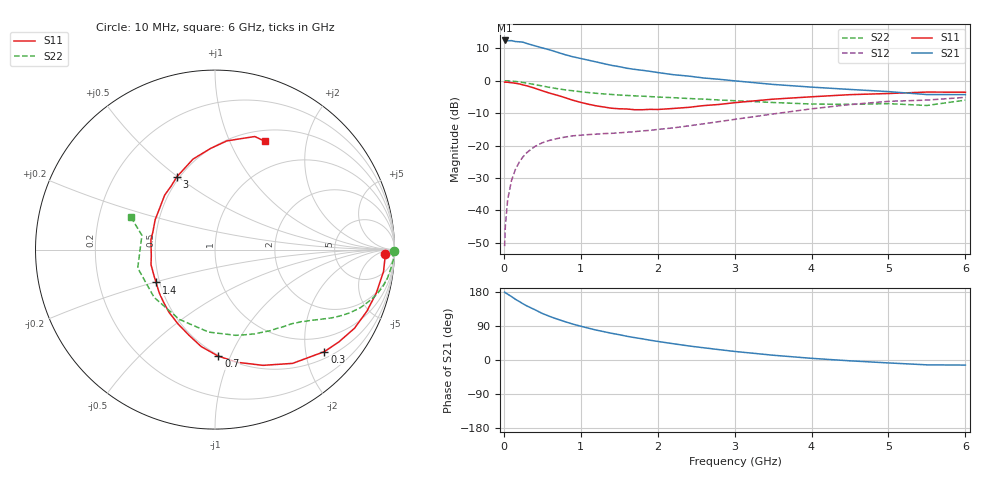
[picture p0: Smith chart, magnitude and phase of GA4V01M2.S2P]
! Infineon Technologies  Discrete & RF Semiconductors
! BF775
! Si NPN RF Bipolar Junction Transistor in SOT23
! VCE = 4 V  IC = 1.2 mA
! Common Emitter S-Parameters:  May  1996
# GHz  S  MA  R  50
!  f  S11  S21  S12  S22
! GHz  MAG  ANG  MAG  ANG  MAG  ANG  MAG  ANG
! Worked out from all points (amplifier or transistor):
!   36 points, 10 MHz to 6 GHz, reference 50 ohm
!   highest |S21| = 12.4 dB at 10 MHz (marker M1)
!   |S21| within 3 dB of that: start of sweep to 609.4 MHz
!   unconditionally stable (mu >= 1): 1.361 GHz to 3.872 GHz; 5.166 GHz to end of sweep
!   at 250 MHz: K = 0.22, MSG = 17.7 dB, |S12| = -23.5 dB
!   at 1.4 GHz: K = 1.03, MAG = 9.5 dB, |S12| = -16.2 dB
!   at 6 GHz: K = 1.01, MAG = -0.2 dB, |S12| = -5.1 dB
!   S11 on the Smith chart (normalised r, x): 10 MHz: 30, -16; 300 MHz: 0.64, -2.39; 700 MHz: 0.49, -0.90; 1.4 GHz: 0.48, -0.20; 3 GHz: 0.48, +0.50; 6 GHz: 0.63, +1.37
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0.01  0.9487 -1.6  4.177 179.1  0.0028 90.2  1 -0.6
0.02  0.948 -3.0  4.107 177.3  0.0058 88.7  0.9902 -1.3
0.05  0.947 -7.4  4.118 173.7  0.0147 85.9  0.9952 -3.2
0.1  0.9304 -15.2  4.153 167.4  0.029 81.0  0.9848 -6.3
0.15  0.9131 -22.1  4.017 160.3  0.0426 75.8  0.9737 -9.5
0.25  0.8608 -36.7  3.925 148.2  0.0671 67.9  0.9378 -15.1
0.3  0.8334 -43.0  3.749 142.6  0.0779 64.4  0.9155 -17.6
0.4  0.7674 -55.7  3.463 133.0  0.0961 58.1  0.8734 -21.7
0.5  0.6985 -67.4  3.207 122.8  0.1103 52.9  0.8288 -25.2
0.6  0.6406 -78.7  2.981 114.7  0.1206 48.4  0.7866 -28.1
0.7  0.5942 -88.2  2.736 107.5  0.1285 44.7  0.7523 -30.4
0.9  0.4982 -107.0  2.336 94.6  0.1413 40.1  0.6985 -33.9
1.1  0.4333 -126.2  2.072 84.0  0.1475 37.6  0.6555 -37.2
1.4  0.376 -150.9  1.725 70.5  0.1541 36.7  0.6132 -41.6
1.9  0.3613 171.3  1.395 52.2  0.1714 39.8  0.5686 -49.7
2.2  0.3726 153.5  1.239 43.0  0.1869 41.9  0.5475 -55.5
3  0.4577 117.7  0.995 22.6  0.253 44.6  0.4914 -76.4
3.5  0.5192 103.6  0.876 12.6  0.3067 42.1  0.4609 -94.4
4.5  0.6091 83.8  0.733 -2.2  0.4291 30.8  0.4312 -141.9
5  0.6345 76.9  0.679 -7.7  0.4801 22.8  0.4426 -166.6
5.5  0.668 70.6  0.611 -12.8  0.5023 13.8  0.4149 168.9
6  0.6641 65.1  0.61 -13.4  0.5536 9.1  0.5012 159.0
